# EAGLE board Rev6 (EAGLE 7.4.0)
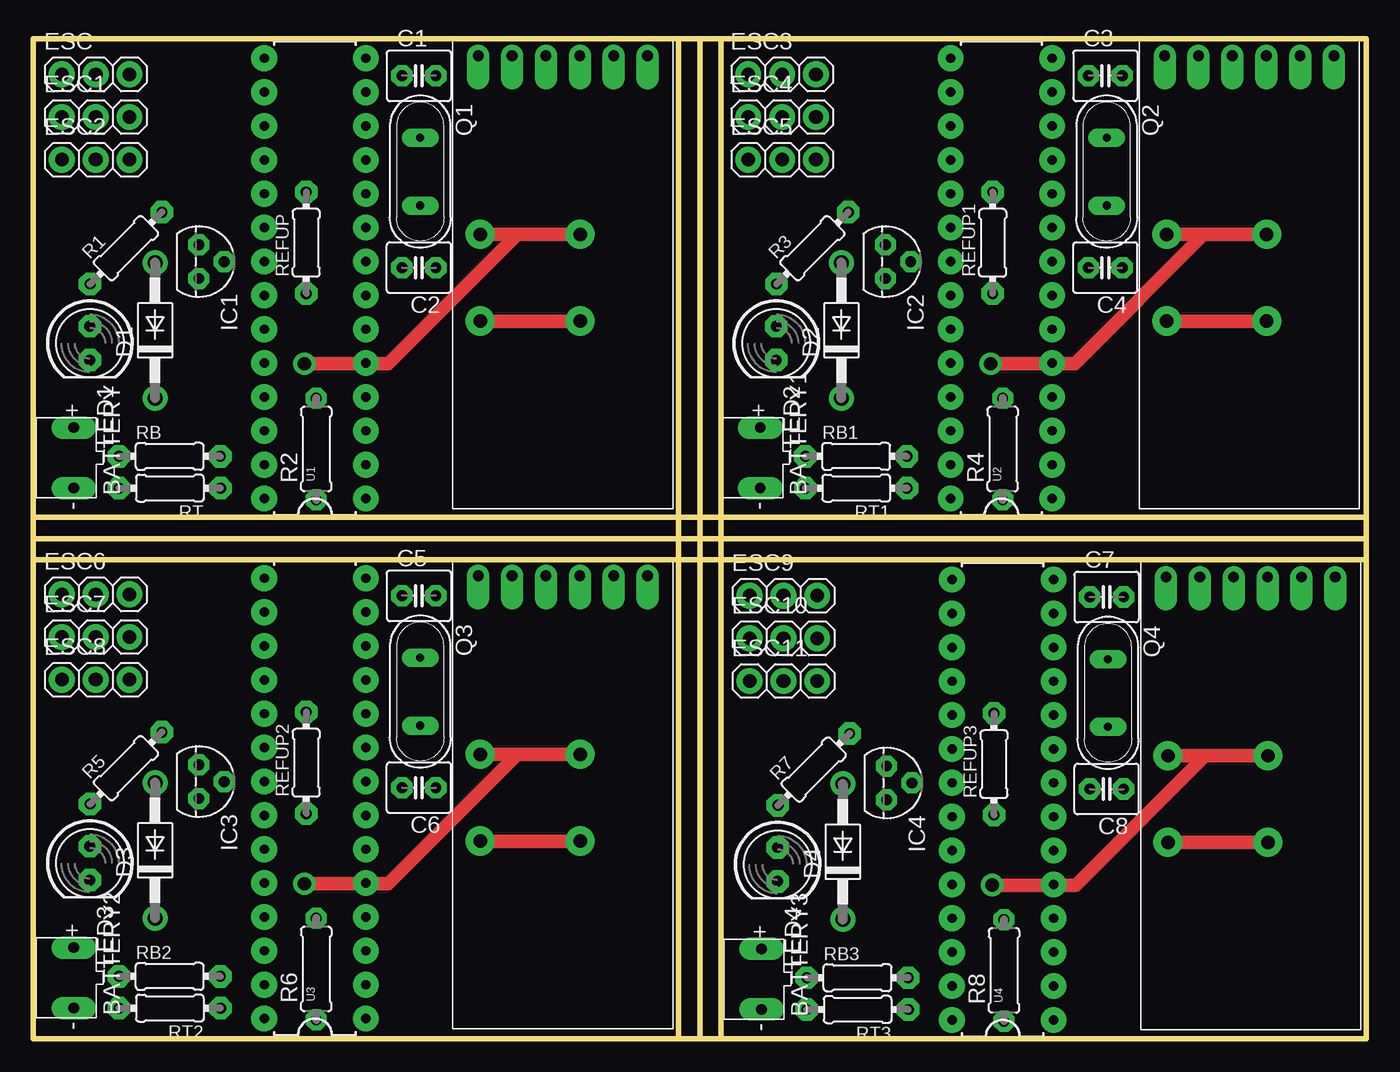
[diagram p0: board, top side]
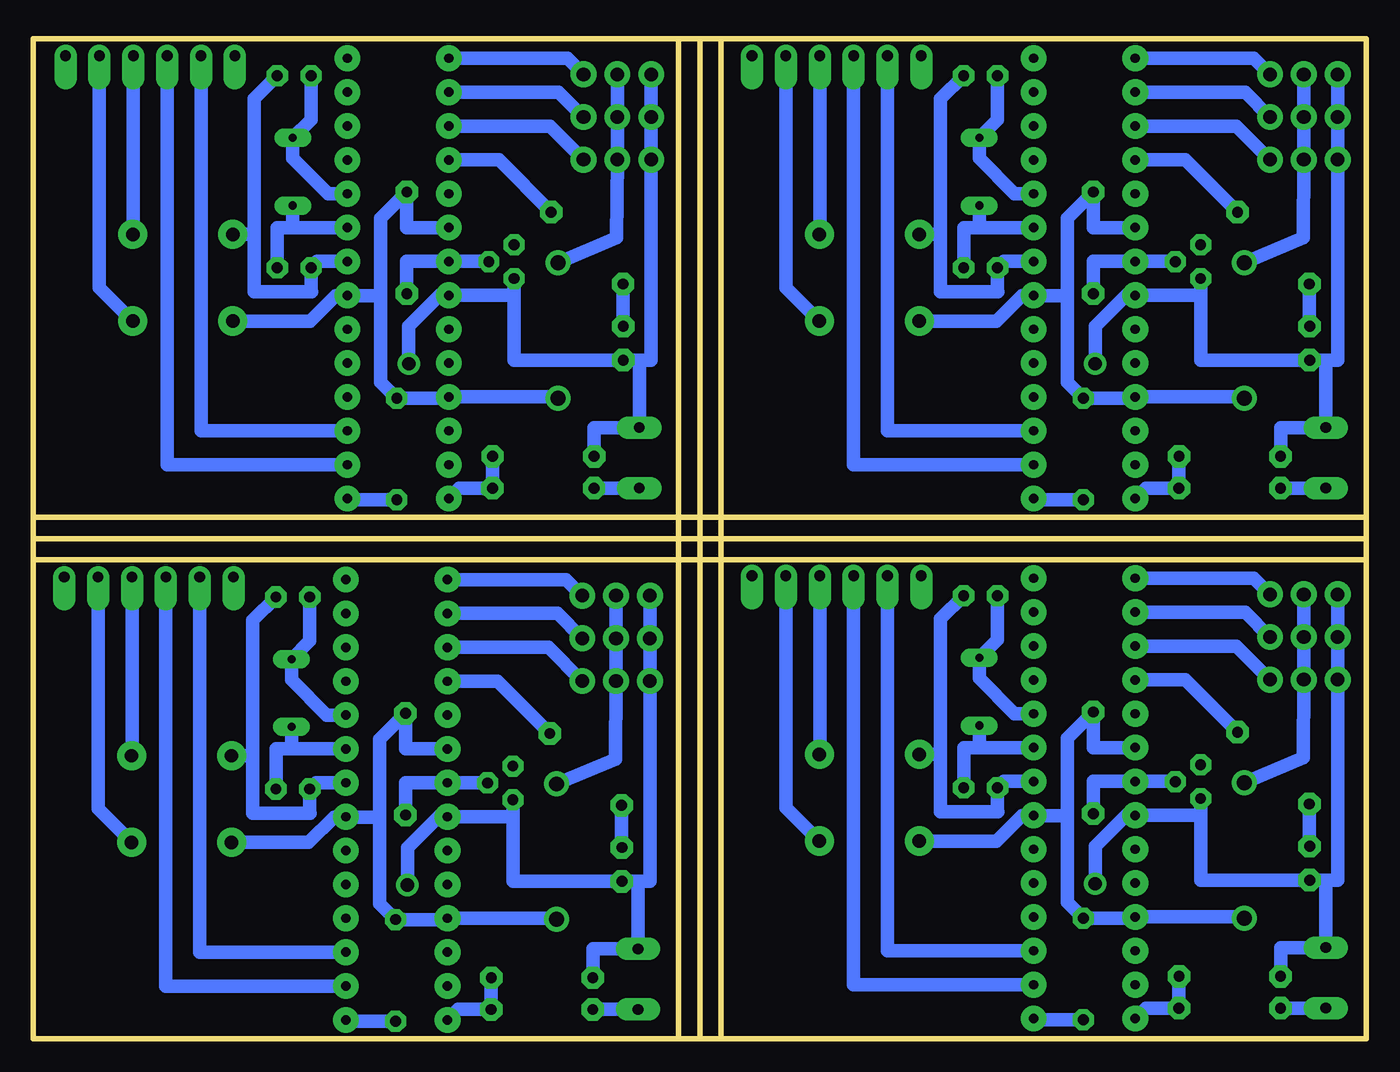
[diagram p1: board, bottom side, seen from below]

Size 100 x 75 mm. Coordinates in mm from the lower left corner, seen from the top.
Outline: 100,35.9 100,0 51.6,0
Outline: 100,35.9 100,37.5
Outline: 100,37.5 100,39.1
Outline: 100,39.1 100,75 51.6,75
Outline: 51.6,75 50,75
Outline: 50,75 48.4,75
Outline: 48.4,75 0,75 0,39
Outline: 48.4,0 0,0 0,35.9
Outline: 48.4,0 50,0
Outline: 50,0 51.6,0
Outline: 0,39 0,37.5
Outline: 0,37.5 0,35.9
Outline: 0,37.5 100,37.5
Outline: 50,0 50,75
Outline: 0,35.9 100,35.9
Outline: 100,39.1 0.1,39.1 0,39
Outline: 51.6,0 51.6,75
Outline: 48.4,75 48.4,0
Copper layers (1*16): Top 0.035mm / dielectric 1.5mm / Bottom 0.035mm
Design rules "default *": minimum track width 10mil, minimum drill 24mil, track to track 15mil, track to pad 15mil, pad to pad 15mil, via to via 15mil, smd to smd 8mil, copper to edge 15mil, drill to drill 8mil, minimum pad ring 15mil, minimum via ring 8mil, stop-mask expansion 4mil, vias tented up to drill 0mil, thermal gap 10mil
Milling: 4 lines

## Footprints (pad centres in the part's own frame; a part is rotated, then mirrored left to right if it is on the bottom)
JST-PH-2-THM = drill 0.8 pad 1.676 long: 1 2.27,0; 2 -2.27,0
C2.5-4 = drill 0.813 pad 1.6 octagon: 1 -1.27,0; 2 1.27,0
DO41-10 = drill 1.118: A 5.08,0; C -5.08,0
1X03 = drill 1.016 pad 1.93: 1 -2.54,0; 2 0,0; 3 2.54,0
TO92 = drill 0.813 octagon: 1 -1.27,0; 2 0,1.905; 3 1.27,0
LED5MM = drill 0.813 pad 1.676 octagon: A -1.27,0; K 1.27,0
QS = drill 0.61 long: 1 -2.54,0; 2 2.54,0
0204/7 = drill 0.813 pad 1.676 octagon: 1 -3.81,0; 2 3.81,0
0207/7 = drill 0.813 octagon: 1 -3.81,0; 2 3.81,0
DIL28-3 = drill 0.7 pad 1.93: 1 -16.51,-3.81; 2 -13.97,-3.81; 3 -11.43,-3.81; 4 -8.89,-3.81; 5 -6.35,-3.81; 6 -3.81,-3.81; 7 -1.27,-3.81; 8 1.27,-3.81; 9 3.81,-3.81; 10 6.35,-3.81; 11 8.89,-3.81; 12 11.43,-3.81; 13 13.97,-3.81; 14 16.51,-3.81; 15 16.51,3.81; 16 13.97,3.81; 17 11.43,3.81; 18 8.89,3.81; 19 6.35,3.81; 20 3.81,3.81; 21 1.27,3.81; 22 -1.27,3.81; 23 -3.81,3.81; 24 -6.35,3.81; 25 -8.89,3.81; 26 -11.43,3.81; 27 -13.97,3.81; 28 -16.51,3.81
HC06 = drill 0.8 pad 1.676 offset: EN -6.35,0; GND -1.27,0; RX 3.81,0; STATE 6.35,0; TX 1.27,0; VCC -3.81,0

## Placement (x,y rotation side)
BATTERY  [JST-PH-2-THM]  3.03,43.56 90 top
BATTERY1  [JST-PH-2-THM]  54.53,43.56 90 top
BATTERY2  [JST-PH-2-THM]  3.03,4.56 90 top
BATTERY3  [JST-PH-2-THM]  54.63,4.46 90 top
C1  [C2.5-4]  28.93,72.22 0 top
C2  [C2.5-4]  28.93,57.82 180 top
C3  [C2.5-4]  80.43,72.22 0 top
C4  [C2.5-4]  80.43,57.82 180 top
C5  [C2.5-4]  28.93,33.22 0 top
C6  [C2.5-4]  28.93,18.82 180 top
C7  [C2.5-4]  80.53,33.12 0 top
C8  [C2.5-4]  80.53,18.72 180 top
D1  1N4933  [DO41-10]  9.13,53.12 90 top
D2  1N4933  [DO41-10]  60.63,53.12 90 top
D3  1N4933  [DO41-10]  9.13,14.12 90 top
D4  1N4933  [DO41-10]  60.73,14.02 90 top
ESC  [1X03]  4.68,72.32 0 top
ESC1  [1X03]  4.68,69.12 0 top
ESC2  [1X03]  4.68,65.92 0 top
ESC3  [1X03]  56.18,72.32 0 top
ESC4  [1X03]  56.18,69.12 0 top
ESC5  [1X03]  56.18,65.92 0 top
ESC6  [1X03]  4.68,33.32 0 top
ESC7  [1X03]  4.68,30.12 0 top
ESC8  [1X03]  4.68,26.92 0 top
ESC9  [1X03]  56.28,33.22 0 top
ESC10  [1X03]  56.28,30.02 0 top
ESC11  [1X03]  56.28,26.82 0 top
IC1  LM336LP  [TO92]  12.42,58.27 270 top
IC2  LM336LP  [TO92]  63.92,58.27 270 top
IC3  LM336LP  [TO92]  12.42,19.27 270 top
IC4  LM336LP  [TO92]  64.02,19.17 270 top
LED1  [LED5MM]  4.24,52.16 270 top
LED2  [LED5MM]  55.74,52.16 270 top
LED3  [LED5MM]  4.24,13.16 270 top
LED4  [LED5MM]  55.84,13.06 270 top
Q1  [QS]  29.03,65.02 270 top
Q2  [QS]  80.53,65.02 270 top
Q3  [QS]  29.03,26.02 270 top
Q4  [QS]  80.63,25.92 270 top
R1  270  [0204/7]  6.96,59.29 45 top
R2  10000  [0207/7]  21.23,44.22 90 top
R3  270  [0204/7]  58.46,59.29 45 top
R4  10000  [0207/7]  72.73,44.22 90 top
R5  270  [0204/7]  6.96,20.29 45 top
R6  10000  [0207/7]  21.23,5.22 90 top
R7  270  [0204/7]  58.56,20.19 45 top
R8  10000  [0207/7]  72.83,5.12 90 top
RB  20000  [0204/7]  10.23,43.67 0 top
RB1  20000  [0204/7]  61.73,43.67 0 top
RB2  20000  [0204/7]  10.23,4.67 0 top
RB3  20000  [0204/7]  61.83,4.57 0 top
REFUP  3300  [0204/7]  20.48,59.69 90 top
REFUP1  3300  [0204/7]  71.98,59.69 90 top
REFUP2  3300  [0204/7]  20.48,20.69 90 top
REFUP3  3300  [0204/7]  72.08,20.59 90 top
RT  220000  [0204/7]  10.24,41.28 180 top
RT1  220000  [0204/7]  61.74,41.28 180 top
RT2  220000  [0204/7]  10.24,2.28 180 top
RT3  220000  [0204/7]  61.84,2.18 180 top
U1  ATMEGA328P_PDIP  [DIL28-3]  21.14,57.02 90 top
U2  ATMEGA328P_PDIP  [DIL28-3]  72.64,57.02 90 top
U3  ATMEGA328P_PDIP  [DIL28-3]  21.14,18.02 90 top
U4  ATMEGA328P_PDIP  [DIL28-3]  72.74,17.92 90 top
U$1  HC06  [HC06]  39.73,73.72 180 top
U$2  HC06  [HC06]  91.23,73.72 180 top
U$3  HC06  [HC06]  39.73,34.72 180 top
U$4  HC06  [HC06]  91.33,34.62 180 top

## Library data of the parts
BATTERY BATTERY1-BATTERY3 LED1-LED4 R1 R3 R5 R7 RB RB1-RB3 REFUP REFUP1-REFUP3 RT RT1-RT3 = adafruit
C1-C8 = capacitor-wima
D1-D4 = diode
ESC ESC1-ESC11 = pinhead
IC1-IC4 = VLADLIBRARY
Q1-Q4 = special
R2 R4 R6 R8 = resistor
U1-U4 = SparkFun-DigitalIC
U$1-U$4 = ccs

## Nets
BUTTON: ESC2.3 U1.17
BUTTON1: ESC5.3 U2.17
BUTTON2: ESC8.3 U3.17
BUTTON3: ESC11.3 U4.17
ESC: ESC.3 U1.15
ESC1: ESC3.3 U2.15
ESC2: ESC6.3 U3.15
ESC3: ESC9.3 U4.15
GND: BATTERY.1 C1.2 C2.2 ESC1.1 ESC2.1 ESC.1 IC1.3 LED1.K RB.1 U1.8 U1.22 U$1.GND
GND1: BATTERY1.1 C3.2 C4.2 ESC3.1 ESC4.1 ESC5.1 IC2.3 LED2.K RB1.1 U2.8 U2.22 U$2.GND
GND2: BATTERY2.1 C5.2 C6.2 ESC6.1 ESC7.1 ESC8.1 IC3.3 LED3.K RB2.1 U3.8 U3.22 U$3.GND
GND3: BATTERY3.1 C7.2 C8.2 ESC9.1 ESC10.1 ESC11.1 IC4.3 LED4.K RB3.1 U4.8 U4.22 U$4.GND
LED: R1.2 U1.18
LED1: R3.2 U2.18
LED2: R5.2 U3.18
LED3: R7.2 U4.18
N$1: BATTERY1.2 RT1.2
N$2: LED1.A R1.1
N$3: C1.1 Q1.1 U1.10
N$4: BATTERY.2 RT.2
N$5: C2.1 Q1.2 U1.9
N$6: LED2.A R3.1
N$7: R2.1 U1.1
N$8: C3.1 Q2.1 U2.10
N$9: C4.1 Q2.2 U2.9
N$10: D1.A ESC1.2 ESC2.2 ESC.2
N$11: R4.1 U2.1
N$12: D2.A ESC3.2 ESC4.2 ESC5.2
N$13: BATTERY2.2 RT2.2
N$14: LED3.A R5.1
N$15: C5.1 Q3.1 U3.10
N$16: C6.1 Q3.2 U3.9
N$17: R6.1 U3.1
N$18: D3.A ESC6.2 ESC7.2 ESC8.2
N$19: BATTERY3.2 RT3.2
N$20: LED4.A R7.1
N$21: C7.1 Q4.1 U4.10
N$22: C8.1 Q4.2 U4.9
N$23: R8.1 U4.1
N$24: D4.A ESC9.2 ESC10.2 ESC11.2
RX: U1.2 U$1.TX
RX1: U2.2 U$2.TX
RX2: U3.2 U$3.TX
RX3: U4.2 U$4.TX
STEER: ESC1.3 U1.16
STEER1: ESC4.3 U2.16
STEER2: ESC7.3 U3.16
STEER3: ESC10.3 U4.16
TX: U1.3 U$1.RX
TX1: U2.3 U$2.RX
TX2: U3.3 U$3.RX
TX3: U4.3 U$4.RX
VCC: D1.C R2.2 REFUP.2 U1.7 U1.20 U1.25 U$1.VCC
VCC1: D2.C R4.2 REFUP1.2 U2.7 U2.20 U2.25 U$2.VCC
VCC2: D3.C R6.2 REFUP2.2 U3.7 U3.20 U3.25 U$3.VCC
VCC3: D4.C R8.2 REFUP3.2 U4.7 U4.20 U4.25 U$4.VCC
VOLTMETER: RB.2 RT.1 U1.28
VOLTMETER1: RB1.2 RT1.1 U2.28
VOLTMETER2: RB2.2 RT2.1 U3.28
VOLTMETER3: RB3.2 RT3.1 U4.28
VREF: IC1.2 REFUP.1 U1.21
VREF1: IC2.2 REFUP1.1 U2.21
VREF2: IC3.2 REFUP2.1 U3.21
VREF3: IC4.2 REFUP3.1 U4.21

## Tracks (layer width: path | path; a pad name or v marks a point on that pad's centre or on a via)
BUTTON
  Bottom 1.016: U1.17 9.75,68.45 ESC2.3
BUTTON1
  Bottom 1.016: U2.17 61.25,68.45 ESC5.3
BUTTON2
  Bottom 1.016: U3.17 9.75,29.45 ESC8.3
BUTTON3
  Bottom 1.016: U4.17 61.35,29.35 ESC11.3
ESC
  Bottom 1.016: U1.15 8.43,73.53 ESC.3
ESC1
  Bottom 1.016: U2.15 59.93,73.53 ESC3.3
ESC2
  Bottom 1.016: U3.15 8.43,34.53 ESC6.3
ESC3
  Bottom 1.016: U4.15 60.03,34.43 ESC9.3
GND  (via drill 1 pad 1.68, 1 pad 2.18)
  Top 1.016: v41.03,60.32 36.33,60.32 | 36.33,60.32 v33.53,60.32 | v20.33,50.62 26.63,50.62 36.33,60.32
  Bottom 1.016: ESC.1 ESC1.1 ESC2.1 2.14,50.89 3.03,50.89 | U1.8 27.19,58.29 C2.2 27.66,56.05 27.63,56.02 31.93,56.02 31.93,60.12 | C1.2 31.93,70.49 31.93,60.12 | U$1.GND 41,60.35 v41.03,60.32 | v33.53,60.32 32.13,60.32 31.93,60.12 | v20.33,50.62 20.33,53.42 18,55.75 U1.22 12.42,55.75 IC1.3 12.42,50.89 LED1.K 3.03,50.89 | RB.1 6.42,45.83 BATTERY.1 3.03,50.89
GND1  (via drill 1 pad 1.68, 1 pad 2.18)
  Top 1.016: v92.53,60.32 87.83,60.32 | 87.83,60.32 v85.03,60.32 | v71.83,50.62 78.13,50.62 87.83,60.32
  Bottom 1.016: ESC3.1 ESC4.1 ESC5.1 53.64,50.89 54.53,50.89 | U2.8 78.69,58.29 C4.2 79.16,56.05 79.13,56.02 83.43,56.02 83.43,60.12 | C3.2 83.43,70.49 83.43,60.12 | U$2.GND 92.5,60.35 v92.53,60.32 | v85.03,60.32 83.63,60.32 83.43,60.12 | v71.83,50.62 71.83,53.42 69.5,55.75 U2.22 63.92,55.75 IC2.3 63.92,50.89 LED2.K 54.53,50.89 | RB1.1 57.92,45.83 BATTERY1.1 54.53,50.89
GND2  (via drill 1 pad 1.68, 1 pad 2.18)
  Top 1.016: v41.03,21.32 36.33,21.32 | 36.33,21.32 v33.53,21.32 | v20.33,11.62 26.63,11.62 36.33,21.32
  Bottom 1.016: ESC6.1 ESC7.1 ESC8.1 2.14,11.89 3.03,11.89 | U3.8 27.19,19.29 C6.2 27.66,17.05 27.63,17.02 31.93,17.02 31.93,21.12 | C5.2 31.93,31.49 31.93,21.12 | U$3.GND 41,21.35 v41.03,21.32 | v33.53,21.32 32.13,21.32 31.93,21.12 | v20.33,11.62 20.33,14.42 18,16.75 U3.22 12.42,16.75 IC3.3 12.42,11.89 LED3.K 3.03,11.89 | RB2.1 6.42,6.83 BATTERY2.1 3.03,11.89
GND3  (via drill 1 pad 1.68, 1 pad 2.18)
  Top 1.016: v92.63,21.22 87.93,21.22 | 87.93,21.22 v85.13,21.22 | v71.93,11.52 78.23,11.52 87.93,21.22
  Bottom 1.016: ESC9.1 ESC10.1 ESC11.1 53.74,11.79 54.63,11.79 | U4.8 78.79,19.19 C8.2 79.26,16.95 79.23,16.92 83.53,16.92 83.53,21.02 | C7.2 83.53,31.39 83.53,21.02 | U$4.GND 92.6,21.25 v92.63,21.22 | v85.13,21.22 83.73,21.22 83.53,21.02 | v71.93,11.52 71.93,14.32 69.6,16.65 U4.22 64.02,16.65 IC4.3 64.02,11.79 LED4.K 54.63,11.79 | RB3.1 58.02,6.73 BATTERY3.1 54.63,11.79
LED
  Bottom 1.016: R1.2 13.57,65.91 U1.18
LED1
  Bottom 1.016: R3.2 65.07,65.91 U2.18
LED2
  Bottom 1.016: R5.2 13.57,26.91 U3.18
LED3
  Bottom 1.016: R7.2 65.17,26.81 U4.18
N$1
  Bottom 1.016: BATTERY1.2 RT1.2
N$2
  Bottom 1.016: LED1.A 4.26,53.43 R1.1
N$3
  Bottom 1.016: U1.10 26.38,63.37 29.03,66.02 Q1.1 27.66,68.93 C1.1
N$4
  Bottom 1.016: BATTERY.2 RT.2
N$5
  Bottom 1.016: Q1.2 29.03,60.83 | 29.03,60.83 U1.9 | C2.1 30.2,60.83 29.03,60.83
N$6
  Bottom 1.016: LED2.A 55.76,53.43 R3.1
N$7
  Bottom 1.016: R2.1 24.85,40.41 U1.1
N$8
  Bottom 1.016: U2.10 77.88,63.37 80.53,66.02 Q2.1 79.16,68.93 C3.1
N$9
  Bottom 1.016: Q2.2 80.53,60.83 | 80.53,60.83 U2.9 | C4.1 81.7,60.83 80.53,60.83
N$10
  Bottom 1.016: D1.A 4.73,60.06 ESC2.2 ESC1.2 ESC.2
N$11
  Bottom 1.016: R4.1 76.35,40.41 U2.1
N$12
  Bottom 1.016: D2.A 56.23,60.06 ESC5.2 ESC4.2 ESC3.2
N$13
  Bottom 1.016: BATTERY2.2 RT2.2
N$14
  Bottom 1.016: LED3.A 4.26,14.43 R5.1
N$15
  Bottom 1.016: U3.10 26.38,24.37 29.03,27.02 Q3.1 27.66,29.93 C5.1
N$16
  Bottom 1.016: Q3.2 29.03,21.83 | 29.03,21.83 U3.9 | C6.1 30.2,21.83 29.03,21.83
N$17
  Bottom 1.016: R6.1 24.85,1.41 U3.1
N$18
  Bottom 1.016: D3.A 4.73,21.06 ESC8.2 ESC7.2 ESC6.2
N$19
  Bottom 1.016: BATTERY3.2 RT3.2
N$20
  Bottom 1.016: LED4.A 55.86,14.33 R7.1
N$21
  Bottom 1.016: U4.10 77.98,24.27 80.63,26.92 Q4.1 79.26,29.83 C7.1
N$22
  Bottom 1.016: Q4.2 80.63,21.73 | 80.63,21.73 U4.9 | C8.1 81.8,21.73 80.63,21.73
N$23
  Bottom 1.016: R8.1 76.45,1.31 U4.1
N$24
  Bottom 1.016: D4.A 56.33,20.96 ESC11.2 ESC10.2 ESC9.2
RX
  Bottom 1.016: U$1.TX 38.46,43.05 U1.2
RX1
  Bottom 1.016: U$2.TX 89.96,43.05 U2.2
RX2
  Bottom 1.016: U$3.TX 38.46,4.05 U3.2
RX3
  Bottom 1.016: U$4.TX 90.06,3.95 U4.2
STEER
  Bottom 1.016: U1.16 9.09,70.99 ESC1.3
STEER1
  Bottom 1.016: U2.16 60.59,70.99 ESC4.3
STEER2
  Bottom 1.016: U3.16 9.09,31.99 ESC7.3
STEER3
  Bottom 1.016: U4.16 60.69,31.89 ESC10.3
TX
  Bottom 1.016: U$1.RX 35.92,45.59 U1.3
TX1
  Bottom 1.016: U$2.RX 87.42,45.59 U2.3
TX2
  Bottom 1.016: U$3.RX 35.92,6.59 U3.3
TX3
  Bottom 1.016: U$4.RX 87.52,6.49 U4.3
VCC  (via drill 1 pad 2.18)
  Top 1.016: v41.03,53.82 v33.53,53.82
  Bottom 1.016: U1.20 20.48,60.83 REFUP.2 22.43,61.54 22.43,55.72 | 22.43,55.72 24.92,55.72 U1.7 24.97,55.72 25.83,55.72 27.73,53.82 v33.53,53.82 | 22.43,55.72 22.43,49.23 R2.2 17.42,48.03 U1.25 9.22,48.13 D1.C | U$1.VCC 43.54,56.33 v41.03,53.82
VCC1  (via drill 1 pad 2.18)
  Top 1.016: v92.53,53.82 v85.03,53.82
  Bottom 1.016: U2.20 71.98,60.83 REFUP1.2 73.93,61.54 73.93,55.72 | 73.93,55.72 76.42,55.72 U2.7 76.47,55.72 77.33,55.72 79.23,53.82 v85.03,53.82 | 73.93,55.72 73.93,49.23 R4.2 68.92,48.03 U2.25 60.72,48.13 D2.C | U$2.VCC 95.04,56.33 v92.53,53.82
VCC2  (via drill 1 pad 2.18)
  Top 1.016: v41.03,14.82 v33.53,14.82
  Bottom 1.016: U3.20 20.48,21.83 REFUP2.2 22.43,22.54 22.43,16.72 | 22.43,16.72 24.92,16.72 U3.7 24.97,16.72 25.83,16.72 27.73,14.82 v33.53,14.82 | 22.43,16.72 22.43,10.23 R6.2 17.42,9.03 U3.25 9.22,9.13 D3.C | U$3.VCC 43.54,17.33 v41.03,14.82
VCC3  (via drill 1 pad 2.18)
  Top 1.016: v92.63,14.72 v85.13,14.72
  Bottom 1.016: U4.20 72.08,21.73 REFUP3.2 74.03,22.44 74.03,16.62 | 74.03,16.62 76.52,16.62 U4.7 76.57,16.62 77.43,16.62 79.33,14.72 v85.13,14.72 | 74.03,16.62 74.03,10.13 R8.2 69.02,8.93 U4.25 60.82,9.03 D4.C | U$4.VCC 95.14,17.23 v92.63,14.72
VOLTMETER
  Bottom 1.016: U1.28 16.55,41.28 RT.1 14.04,41.29 RB.2
VOLTMETER1
  Bottom 1.016: U2.28 68.05,41.28 RT1.1 65.54,41.29 RB1.2
VOLTMETER2
  Bottom 1.016: U3.28 16.55,2.28 RT2.1 14.04,2.29 RB2.2
VOLTMETER3
  Bottom 1.016: U4.28 68.15,2.18 RT3.1 65.64,2.19 RB3.2
VREF
  Bottom 1.016: IC1.2 14.34,58.29 U1.21 20.48,58.29 REFUP.1
VREF1
  Bottom 1.016: IC2.2 65.84,58.29 U2.21 71.98,58.29 REFUP1.1
VREF2
  Bottom 1.016: IC3.2 14.34,19.29 U3.21 20.48,19.29 REFUP2.1
VREF3
  Bottom 1.016: IC4.2 65.94,19.19 U4.21 72.08,19.19 REFUP3.1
